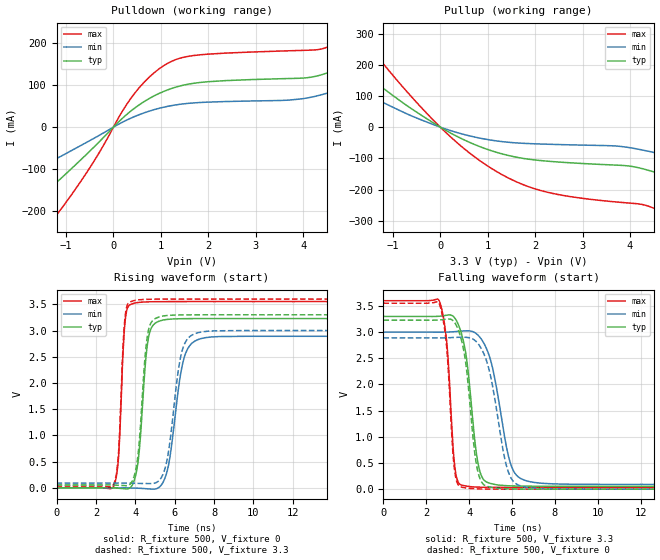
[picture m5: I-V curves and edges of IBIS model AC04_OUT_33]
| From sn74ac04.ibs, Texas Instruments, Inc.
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[Model]   AC04_OUT_33
Model_type  Output
Vref =   0
Rref =   500
Cref =   50p
Vmeas =   1.65
| variable   typ   min   max
C_comp   10.64pF   6.97pF   15.36pF
| C_pullup   10.40pF   6.99pF   12.98pF
| C_pulldown   10.88pF   6.97pF   15.36pF
[Temperature Range]   40   100   -40
| Ambient temperature   25   85   -40
[Voltage range]   3.3   3   3.6
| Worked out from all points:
|   slope of the pulldown table from 0 to 0.495 V, typ, clamps not added: 10 ohm
|   slope of the pullup table from 0 to 0.495 V, typ, clamps not added: 12.3 ohm
|   rising waveform, R_fixture 500, V_fixture 0: 20-80 % time 383ps typ, 617ps min, 246ps max; typ from 0 V to 3.23 V
|   falling waveform, R_fixture 500, V_fixture 3.3: 20-80 % time 513ps typ, 782ps min, 325ps max; typ from 3.3 V to 0.055 V
|   rising waveform, R_fixture 500, V_fixture 3.3: 20-80 % time 374ps typ, 581ps min, 244ps max; typ from 0.055 V to 3.3 V
|   falling waveform, R_fixture 500, V_fixture 0: 20-80 % time 500ps typ, 754ps min, 320ps max; typ from 3.23 V to 0 V
[Pulldown]
| AC04_OUT_33
|   Voltage   I(typ)   I(min)   I(max)
-5V       -469.8mA   -290.4mA   -597.1mA
-4.245V   -407.3mA   -249mA     -526.2mA
-2.25V    -235.7mA   -137.3mA   -339.5mA
-1.48V    -160.7mA   -92.13mA   -249.5mA
-690mV    -78.28mA   -44.02mA   -129.9mA
520mV     51.46mA    28.76mA    91.09mA
1.4V      98.27mA    54.57mA    164.8mA
4.34V     123.7mA    76.06mA    185.7mA
5.19V     165.4mA    109.2mA    239.8mA
6.26V     245.5mA    168mA      355.3mA
7.385V    349.5mA    242.1mA    505.1mA
10V       641.4mA    437.7mA    934.9mA
[Pullup]
| AC04_OUT_33
|   Voltage   I(typ)   I(min)   I(max)
-5V       610.9mA    379.3mA    1.028A
-4.31V    515.1mA    323.5mA    856mA
-2.865V   325.1mA    207.5mA    530.1mA
-1.89V    204.9mA    130.9mA    332.8mA
365mV     -30.68mA   -17.89mA   -51.37mA
1.25V     -83.54mA   -45.44mA   -147.9mA
2.105V    -107mA     -54.02mA   -202.7mA
4.32V     -135.5mA   -75.13mA   -250.1mA
5.35V     -190.9mA   -113.9mA   -324.2mA
7.15V     -315.7mA   -196.9mA   -479mA
9.57V     -503mA     -320.5mA   -697.4mA
10V       -537.8mA   -343.4mA   -737.4mA
[Ramp]
| AC04_OUT_33
| variable   typ   min   max
dV/dt_r   1.95/3.95E-10   1.75/6.26E-10   2.14/2.57E-10
dV/dt_f   1.96/5.26E-10   1.76/7.96E-10   2.16/3.36E-10
R_load = 500
[Rising Waveform]
| AC04_OUT_33
R_fixture =   500
C_fixture =   0
L_fixture =   0
V_fixture =   0
V_fixture_min = 0
V_fixture_max = 0
|   Time   V(typ)   V(min)   V(max)
0s        1.117nV    1.975nV    631.8pV
2.935ns   -3.094mV   361.3uV    56.91mV
3.15ns    -8.305mV   314.1uV    585.7mV
3.495ns   -19.65mV   -294.9uV   3.221V
4.02ns    240.1mV    -5.925mV   3.527V
4.67ns    2.864V     -20.33mV   3.547V
5.475ns   3.204V     156.1mV    3.551V
6.48ns    3.226V     2.48V      3.552V
7.55ns    3.228V     2.863V     3.552V
50ns      3.228V     2.89V      3.552V
[Falling Waveform]
| AC04_OUT_33
R_fixture =   500
C_fixture =   0
L_fixture =   0
V_fixture =   3.3
V_fixture_min = 3
V_fixture_max = 3.6
|   Time   V(typ)   V(min)   V(max)
0s        3.3V       3V         3.6V
2.61ns    3.304V     2.999V     3.593V
2.945ns   3.323V     3.001V     2.849V
3.365ns   3.248V     3.01V      325.8mV
3.88ns    2.488V     3.025V     58.13mV
4.32ns    737.4mV    2.975V     40.52mV
4.605ns   226.5mV    2.843V     36.78mV
5.965ns   62.68mV    447.5mV    33.18mV
7ns       56.57mV    130mV      32.98mV
50ns      55.35mV    90.5mV     32.95mV
[Rising Waveform]
| AC04_OUT_33
R_fixture =   500
C_fixture =   0
L_fixture =   0
V_fixture =   3.3
V_fixture_min = 3
V_fixture_max = 3.6
|   Time   V(typ)   V(min)   V(max)
0s        55.35mV    90.5mV     32.95mV
2.925ns   52.45mV    90.69mV    88.26mV
3.145ns   48.13mV    90.54mV    635.9mV
3.49ns    41.45mV    89.87mV    3.292V
4ns       304.7mV    85.73mV    3.575V
4.63ns    2.93V      81.05mV    3.595V
5.405ns   3.276V     257.2mV    3.599V
6.375ns   3.298V     2.609V     3.6V
7.375ns   3.3V       2.974V     3.6V
50ns      3.3V       3V         3.6V
[Falling Waveform]
| AC04_OUT_33
R_fixture =   500
C_fixture =   0
L_fixture =   0
V_fixture =   0
V_fixture_min = 0
V_fixture_max = 0
|   Time   V(typ)   V(min)   V(max)
0s        3.228V     2.89V      3.552V
2.61ns    3.232V     2.89V      3.538V
2.945ns   3.248V     2.892V     2.744V
3.315ns   3.188V     2.898V     377.7mV
3.7ns     2.745V     2.902V     33.18mV
4.525ns   180.7mV    2.715V     4.052mV
4.98ns    39.24mV    2.193V     1.52mV
5.81ns    6.31mV     349.8mV    304.3uV
6.72ns    1.161mV    33.89mV    58.89uV
50ns      -135.8pV   -5.359nV   -3.057nV
